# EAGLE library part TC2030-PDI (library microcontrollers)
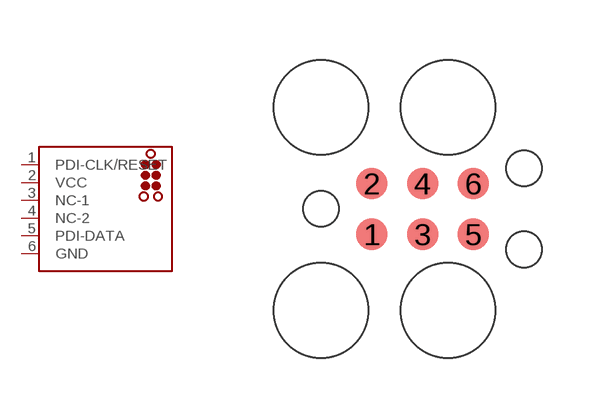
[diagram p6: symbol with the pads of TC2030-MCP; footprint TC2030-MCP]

Designator prefix -

## TC2030-PDI  [TC2030-MCP]
1  PDI-CLK/RESET  pas
2  VCC  pwr
3  NC-1  pwr
4  NC-2
5  PDI-DATA  out
6  GND

## Footprint TC2030-MCP (pad centres in mm)
TAG-CONNECT ICSP Connector - Legged version Manufacturer: Tag-Connect Cable for easy In-Circuit Serial Programming. Designed for Microchip ICD2, suitable for many others. NOTE: Eagle's default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
smd 0.787 x 0.787: 1 1.27,-0.635; 2 1.27,0.635; 3 2.54,-0.635; 4 2.54,0.635; 5 3.81,-0.635; 6 3.81,0.635
hole 0.889 at 0,0
hole 0.889 at 5.08,-1.016
hole 0.889 at 5.08,1.016
hole 2.375 at 0,2.54
hole 2.375 at 0,-2.54
hole 2.375 at 3.175,-2.54
hole 2.375 at 3.175,2.54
